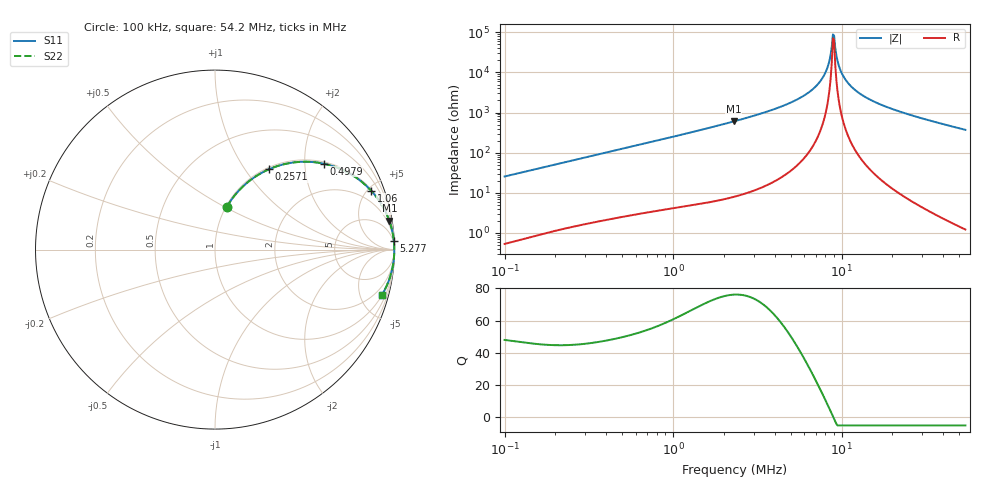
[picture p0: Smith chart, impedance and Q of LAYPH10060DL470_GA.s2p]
! LAYPH10060DL470_GA  S-PARAMETER MODEL  ( General Type )
! Model Generated by TAIYO YUDEN Corporation (http://www.ty-top.com)
! Version 3.0
! TAIYO YUDEN Control No. 180828NI43SB-FBB
! Copyright(c) 2017 TAIYO YUDEN CO.,LTD. All Rights Reserved.
! Product Description (link to TY-COMPAS)
! https://ds.yuden.co.jp/TYCOMPAS/or/detail?pn=LAYPH10060DL470MGA&u=M
! Products Name : Inductors
! Characteristics :
!  Inductance : 47 uH , SRF(min) : -Hz , DC Resistance(max) : 0.098 Ohm
!  Rated Current : Saturation :2.1 A , Temp Rise : 1.4 A (25 degC)
!  Case Size : 10.1 x 10.0 / 0.398 x 0.394 [mm/inch] , Thickness : 6 / 0.236 [mm/inch]
!  (Conditions: Temperature = 25 degC , DC Bias Current/Voltage = 0A / 0V)
! External Node Assignments :
!  1  o---GGG---o  2
! GND o---------o GND
! Frequency Range : 0.1MHz  -  54.20166MHz  [ 402 STEP ]
# MHz S RI R 50
! Freq[MHz].  S11 Real  S11 Imag  S21 Real  S21 Imag  S12 Real  S12 Imag  S22 Real  S22 Imag
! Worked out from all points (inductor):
!   401 points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, 100 kHz to 54.2 MHz, reference 50 ohm
!   read as one part in series: L = 40.5 uH near 103.2 kHz
!   highest Q = 76.1 at 2.292 MHz (marker M1), where L = 41.8 uH
!   self-resonance near 8.871 MHz
!   S11 on the Smith chart (normalised r, x): 100 kHz: 1.01, +0.51; 257.1 kHz: 1.03, +1.29; 497.9 kHz: 1.05, +2.49; 1.06 MHz: 1.09, +5.30; 5.277 MHz: 2, +40; 54.2 MHz: 1.02, -7.42
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0.1  0.0654 0.2371  0.9346 -0.2371  0.9346 -0.2371  0.0654 0.2371
0.2571  0.2992 0.4469  0.7008 -0.4469  0.7008 -0.4469  0.2992 0.4469
0.287043  0.3455 0.4646  0.6545 -0.4646  0.6545 -0.4646  0.3455 0.4646
0.497936  0.6052 0.4789  0.3948 -0.4789  0.3948 -0.4789  0.6052 0.4789
0.823937  0.8044 0.388  0.1956 -0.388  0.1956 -0.388  0.8044 0.388
1.059875  0.8716 0.3266  0.1284 -0.3266  0.1284 -0.3266  0.8716 0.3266
2.291771  0.9712 0.1609  0.0288 -0.1609  0.0288 -0.1609  0.9712 0.1609
2.328125  0.9721 0.1582  0.0279 -0.1582  0.0279 -0.1582  0.9721 0.1582
5.277496  0.9964 0.0501  0.00361 -0.0501  0.00361 -0.0501  0.9964 0.0501
6.682722  0.9983 0.0268  0.00171 -0.0268  0.00171 -0.0268  0.9983 0.0268
7.94582  0.9989 0.0107  0.00105 -0.0107  0.00105 -0.0107  0.9989 0.0107
8.329978  0.999 0.0064  0.000968 -0.0064  0.000968 -0.0064  0.999 0.0064
8.732708  0.9991 0.0021  0.000922 -0.0021  0.000922 -0.0021  0.9991 0.0021
9.011955  0.9991 -0.000773  0.000912 0.000773  0.000912 0.000773  0.9991 -0.000773
9.154909  0.9991 -0.00221  0.000913 0.00221  0.000913 0.00221  0.9991 -0.00221
9.447656  0.9991 -0.00508  0.000929 0.00508  0.000929 0.00508  0.9991 -0.00508
9.749765  0.999 -0.00795  0.000961 0.00795  0.000961 0.00795  0.999 -0.00795
10.22114  0.999 -0.0123  0.00104 0.0123  0.00104 0.0123  0.999 -0.0123
11.05795  0.9987 -0.0196  0.00126 0.0196  0.00126 0.0196  0.9987 -0.0196
13.78367  0.9975 -0.0407  0.00252 0.0407  0.00252 0.0407  0.9975 -0.0407
19.18229  0.9933 -0.0762  0.00668 0.0762  0.00668 0.0762  0.9933 -0.0762
54.20166  0.9316 -0.2508  0.0684 0.2508  0.0684 0.2508  0.9316 -0.2508
